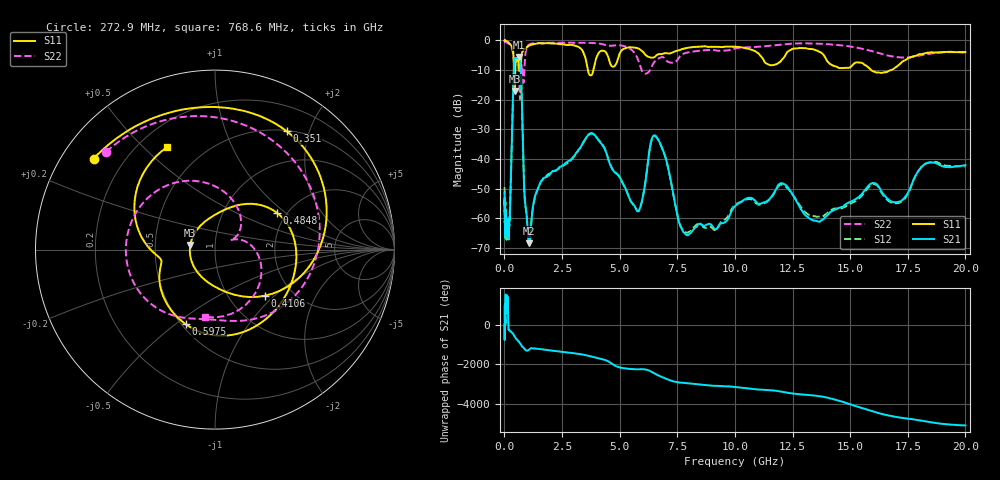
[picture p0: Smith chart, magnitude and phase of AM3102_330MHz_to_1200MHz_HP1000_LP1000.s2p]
! Date/Time: Tue, Sep 11, 2018 5:17 PM
! Network Analyzer: Agilent Technologies E8362B Rev: A.07.50.63
! Sweep from 0.010 to 20.000 GHz, 1601 Points, Sweep Type: LOG
! Power Supply: 4.949 V, 0.001 A
# Hz S DB R 50
!freq MagS11 AngS11 MagS21 AngS21 MagS12 AngS12 MagS22 AngS22
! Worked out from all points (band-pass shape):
!   1601 points, 10 MHz to 20 GHz, reference 50 ohm
!   highest |S21| = -5.61 dB at 617.7 MHz (marker M1); lowest = -68.4 dB at 1.062 GHz (marker M2)
!   |S21| within 3 dB of the highest: 417.4 MHz to 699.8 MHz (282.3 MHz wide, 50.5 % of centre)
!   lowest |S11| = -17.1 dB at 440.9 MHz (marker M3), VSWR 1.33, Z = 37.8 + j1.98 ohm
!   |S11| at or under -10 dB: 415.3 MHz to 469.7 MHz (54.44 MHz wide, 12.3 % of centre); 3.626 GHz to 3.861 GHz (234.3 MHz wide, 6.26 % of centre); 15.91 GHz to 16.77 GHz (859.9 MHz wide, 5.26 % of centre)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
!   |S22| runs from -19.9 to -0.2 dB; largest |S21 - S12| = 0.0099
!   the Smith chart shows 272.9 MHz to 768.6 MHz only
!   S11 on the Smith chart (normalised r, x): 272.9 MHz: 0.09, +0.33; 351 MHz: 0.51, +1.66; 410.6 MHz: 1.46, -0.88; 484.8 MHz: 1.79, +0.87; 597.5 MHz: 0.53, -0.55; 768.6 MHz: 0.31, +0.59
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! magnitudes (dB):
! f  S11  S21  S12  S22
! 10 MHz  0.0  -51.4  -49.5  -0.3
! 35.55 MHz  0.0  -62.2  -63.5  -0.4
! 126.4 MHz  -0.4  -62.5  -63.3  -0.8
! 191.1 MHz  -0.8  -67.1  -65.1  -1.1
! 272.9 MHz  -1.5  -49.3  -49.3  -1.8
! 351 MHz  -2.3  -25.6  -25.7  -3.5
! 410.6 MHz  -8.4  -9.7  -9.8  -6.6
! 440.9 MHz  -17.1  -6.4  -6.4  -8.2
! 447.2 MHz  -16.5  -6.1  -6.2  -8.1
! 484.8 MHz  -7.9  -5.9  -6.0  -6.6
! 597.5 MHz  -7.0  -5.7  -5.8  -8.2
! 617.7 MHz  -7.9  -5.6  -5.7  -10.0
! 682.6 MHz  -10.1  -7.1  -7.1  -19.9
! 768.6 MHz  -4.0  -23.1  -23.2  -8.4
! 869.7 MHz  -2.9  -51.4  -51.9  -10.1
! 1.062 GHz  -1.8  -68.4  -68.6  -1.5
! 1.59 GHz  -1.0  -47.5  -47.6  -0.8
! 3.811 GHz  -11.3  -31.4  -31.3  -0.9
! 5.652 GHz  -2.4  -55.9  -56.1  -4.3
! 6.549 GHz  -5.4  -32.1  -32.3  -6.8
! 7.958 GHz  -2.5  -65.7  -64.8  -4.1
! 20 GHz  -3.9  -42.0  -42.5  -4.0
